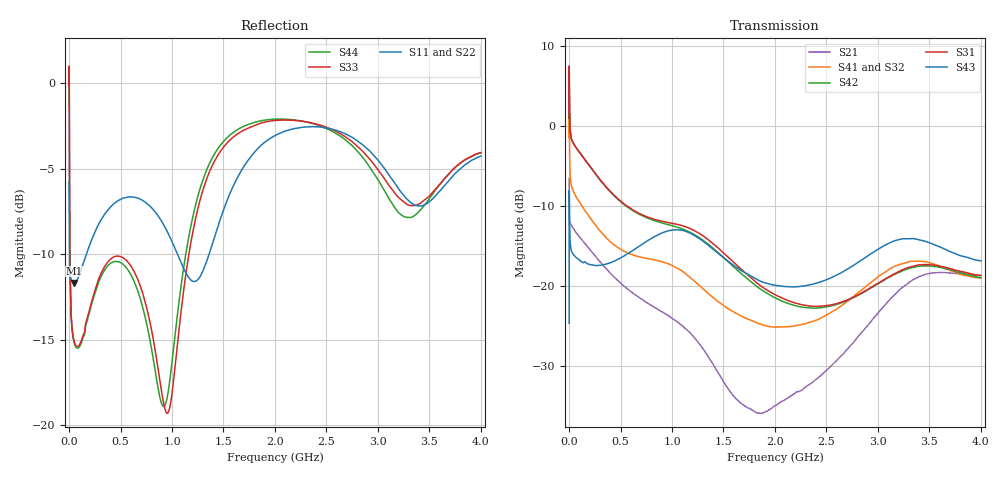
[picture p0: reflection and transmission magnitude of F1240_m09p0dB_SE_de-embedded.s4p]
! Integrated Device Technology
! Corporate Headquarters
! 6024 Silver Creek Valley Road
! San Jose, CA 95138  USA
! Phone:  1-408-284-8200
! Toll Free:  1-800-223-1366
! Webpage:  http://www.idt.com/
! Timing and RF Division
! 515 Groton Road, Suite 102
! Westford, MA 01886-6024
! Device:  F1240
! Description: Dual Intermediate Frequency Digital Variable Gain Amplifier
! Frequency:  10.0 -  500.00 MHz
! Package:  5x5 mm QFN Plastic Package: 32 pin
! Ports:  8 RF, 20 DC
!  Pin  1  = GA3 / Data  Pin 17  = RF OUT_B+
!  Pin  2  = GA4 / CLK  Pin 18  = RF OUT_B-
!  Pin  3  = GA5  Pin 19  = STBY_B
!  Pin  4  = VMODE  Pin 20  = Ground
!  Pin  5  = No Connect  Pin 21  = Ground
!  Pin  6  = GB5  Pin 22  = STB_A
!  Pin  7  = GB4  Pin 23  = RF OUT_A-  = Port 4
!  Pin  8  = GB3  Pin 24  = RF OUT_A+  = Port 3
!  Pin  9  = GB2  Pin 25  = GA0
!  Pin 10  = GB1  Pin 26  = ISET_A
!  Pin 11  = RF IN_B+  Pin 27  = VCC
!  Pin 12  = RF IN_B-  Pin 28  = Ground
!  Pin 13  = Ground  Pin 29  = RF IN_A-  = Port 2
!  Pin 14  = VCC  Pin 30  = RF IN_A+  = Port 1
!  Pin 15  = ISET_B  Pin 31  = GA1
!  Pin 16  = GB0  Pin 32  = GA2 / CSb
! Gain  = +19.5 dB
! State  = 1
! Voltage  = +5.00 V
! Current  = 85.292 mA (one channel only)
! Temperture  =  +25 C
! Test Date  =  2017-10-18
! Board  =  EB4031
! Data:  The device was measured on a custom evaluation board which has
!  individual transmission lines to the RF pins.  Data was collected
!  using a calibrated network analyzer.  The evaluation board was
!  de-embedded using Automatic Fixture Removal.
!  The reference plane is the edge of the package pin.
!  Only Channel A was measured.
!  This data is in single-ended operation.  If your needs are balanced
!  or differential S-parameters then this file needs to be used a
!  linear simulator.
! File Date:  2017-11-10  MJV
! Note:
!  Integrated Device Technology supplies this data as a sample of measured
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# Hz S dB R 100
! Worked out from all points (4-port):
!   410 points, 500 kHz to 4 GHz, reference 100 ohm
!   strongest paths, dB at 500 kHz, 930 MHz, 1.96 GHz, 2.98 GHz, 4 GHz:
!     S43: -24.6, -13.2, -19.8, -15.6, -16.8
!     S31: 1.0, -11.9, -20.8, -19.8, -18.6
!     S42: 1.0, -12.2, -21.2, -19.8, -18.9
!     S41: -1.4, -17.0, -25.0, -19.1, -18.9
!     S32: -1.4, -17.2, -24.9, -19.3, -19.2
!     S21: -6.5, -23.4, -35.3, -23.7, -18.7
!   lowest |S11| = -11.7 dB at 50 MHz (marker M1), VSWR 1.70, Z = 144 - j47.4 ohm
!   |S11| at or under -10 dB: 2.934 MHz to 169.1 MHz (166.1 MHz wide, 193 % of centre); 1.053 GHz to 1.361 GHz (307.9 MHz wide, 25.5 % of centre)
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500000  -5.74 -5.6  -6.49 -5.8  -31.71 77.3  -34.24 76.4
        -6.49 -5.8  -5.74 -5.6  -34.21 75.3  -31.71 78.5
        0.97 -111.2  -1.42 -113.0  -0.11 -0.1  -24.61 -38.0
        -1.43 -111.8  0.97 -110.1  -24.61 -38.1  -0.11 2.2
3500000  -10.43 -20.4  -11.43 -18.6  -24.76 4.7  -29.55 -11.4
         -11.43 -18.6  -10.43 -20.5  -29.51 -11.6  -24.76 4.9
         3.61 156.0  -0.81 141.4  -4.09 -81.6  -10.09 178.0
         -0.84 141.5  3.62 156.2  -10.09 177.9  -4.13 -81.6
5e7  -11.70 -36.1  -12.96 -22.4  -26.13 -17.6  -32.61 -20.7
     -12.96 -22.4  -11.66 -36.6  -32.62 -20.6  -26.10 -17.6
     -2.33 151.5  -8.38 143.2  -15.13 -161.9  -16.18 153.2
     -8.37 143.2  -2.27 151.4  -16.15 153.2  -15.20 -162.5
4.9e8  -6.83 -141.8  -19.47 -122.0  -29.90 -99.4  -37.28 -91.1
       -19.47 -121.9  -6.77 -142.6  -37.40 -88.9  -30.19 -99.4
       -9.24 31.3  -15.39 -11.6  -10.13 -171.3  -16.59 18.5
       -15.29 -12.8  -9.30 29.7  -16.52 18.2  -10.47 -172.0
2.06e9  -2.89 -179.0  -34.29 60.1  -33.39 -20.3  -35.60 0.8
        -34.42 60.4  -2.80 -179.5  -36.18 7.2  -34.87 -13.8
        -21.40 62.7  -24.98 -3.5  -2.16 175.0  -20.20 32.5
        -25.07 -10.5  -21.79 65.5  -19.98 33.7  -2.09 171.9
2.92e9  -3.96 100.7  -24.59 -25.1  -28.87 -153.6  -31.21 -139.6
        -24.60 -25.1  -3.75 101.5  -31.72 -126.7  -30.27 -145.1
        -20.25 -68.5  -19.89 -148.0  -4.44 92.5  -16.80 -94.3
        -19.63 -159.6  -20.29 -65.4  -16.04 -92.1  -4.90 84.9
4e9  -4.26 -127.3  -18.67 122.3  -27.34 -22.0  -28.37 -7.0
     -18.67 122.3  -4.02 -126.0  -28.96 6.4  -29.13 -11.5
     -18.64 56.8  -19.20 -38.1  -4.06 -133.0  -18.25 61.6
     -18.93 -52.1  -18.94 63.1  -16.82 55.5  -4.07 -143.0
